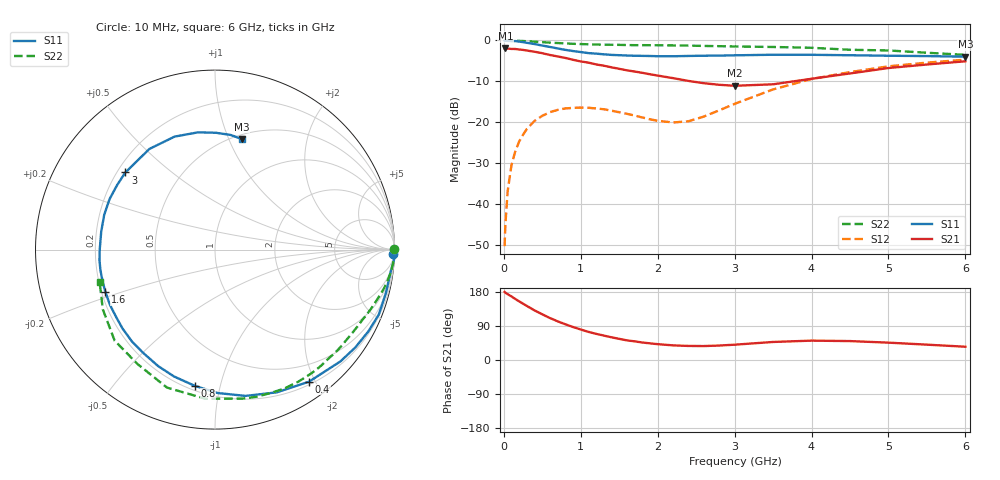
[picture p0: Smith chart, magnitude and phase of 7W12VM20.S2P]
! Infineon Technologies  Discrete & RF Semiconductors
! BFS17W
! Si NPN RF Bipolar Junction Transistor in SOT323
! VCE = 12 V  IC = 0.2 mA
! Common Emitter S-Parameters:  August  1999
# GHz  S  MA  R  50
!  f  S11  S21  S12  S22
! GHz  MAG  ANG  MAG  ANG  MAG  ANG  MAG  ANG
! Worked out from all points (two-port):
!   36 points, 10 MHz to 6 GHz, reference 50 ohm
!   highest |S21| = -1.96 dB at 20 MHz (marker M1); lowest = -11.1 dB at 3 GHz (marker M2)
!   |S21| within 3 dB of the highest: start of sweep to 961.2 MHz
!   lowest |S11| = -4.0 dB at 6 GHz (marker M3), VSWR 4.46, Z = 27.1 + j55.7 ohm
!   |S11| at or under -10 dB: nowhere
!   |S22| runs from -3.5 to 0.0 dB; largest |S21 - S12| = 0.8
!   S11 on the Smith chart (normalised r, x): 10 MHz: 31, -76; 400 MHz: 0.24, -1.92; 800 MHz: 0.23, -0.84; 1.6 GHz: 0.22, -0.18; 3 GHz: 0.23, +0.35; 6 GHz: 0.54, +1.11
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0.01  0.9908 -1.3  0.795 179.5  0.0031 80.8  0.9999 0.2
0.02  0.9999 -3.0  0.798 177.6  0.0057 89.9  0.995 -0.6
0.05  0.9863 -7.1  0.796 173.6  0.0146 87.5  0.9987 -1.7
0.1  0.9827 -14.0  0.788 167.6  0.0305 81.7  0.9987 -3.4
0.15  0.9817 -21.7  0.787 160.9  0.0448 76.2  0.9925 -5.1
0.25  0.9531 -34.9  0.767 148.6  0.0709 68.2  0.9836 -8.4
0.4  0.9034 -54.5  0.728 130.8  0.1046 57.0  0.9661 -12.9
0.6  0.8327 -78.2  0.665 110.7  0.1335 44.8  0.9407 -18.1
0.8  0.7675 -98.4  0.612 94.2  0.1483 35.1  0.9197 -23.1
1.1  0.7012 -124.7  0.536 74.2  0.151 25.2  0.8975 -30.1
1.3  0.6774 -139.5  0.492 64.4  0.1449 21.2  0.8878 -34.9
1.6  0.6547 -158.8  0.432 51.8  0.1274 19.5  0.8791 -42.0
1.9  0.6463 -174.8  0.387 43.9  0.1092 25.8  0.8753 -49.8
2.2  0.6418 171.1  0.347 38.6  0.0999 40.6  0.8701 -57.6
2.4  0.6471 162.5  0.321 37.1  0.1034 53.2  0.8654 -63.2
3  0.6589 139.3  0.28 40.4  0.1685 75.0  0.8445 -79.4
3.5  0.6695 123.1  0.292 47.6  0.2529 75.5  0.8327 -93.7
4  0.6685 109.7  0.341 51.1  0.3387 69.4  0.814 -109.2
4.5  0.6602 98.3  0.396 49.9  0.4115 61.6  0.7699 -124.1
5  0.651 89.6  0.461 45.8  0.4834 53.8  0.7549 -137.8
5.5  0.6447 82.2  0.509 40.5  0.5366 45.9  0.7081 -152.0
6  0.6337 76.5  0.557 35.0  0.5828 38.7  0.6676 -164.3
